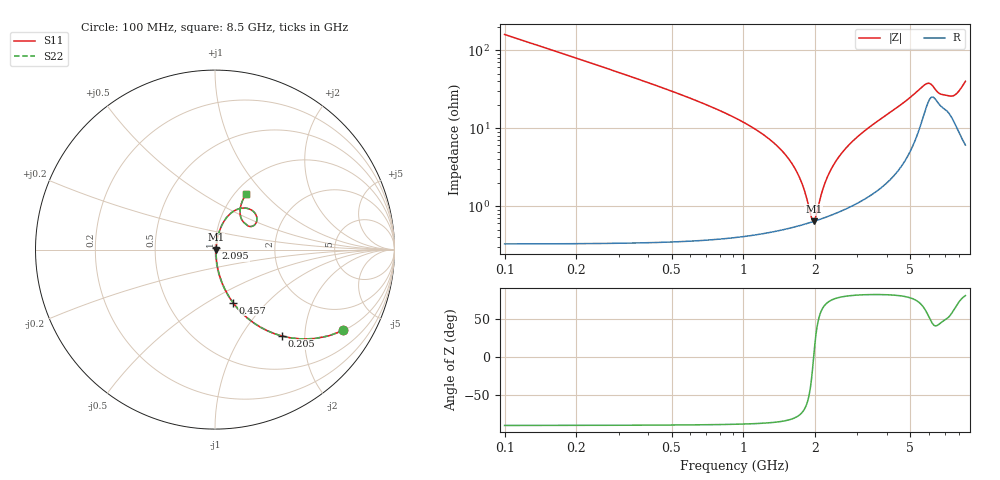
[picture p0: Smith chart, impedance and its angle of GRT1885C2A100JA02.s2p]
!Murata Part Number: GRT1885C2A100JA02
!These Parameters are Measured in Series Mode Connection
!Data Generated on Jun 19, 2026
!  o--ll--o
!Port1  Port2
!  o------o
!Operation Temp=25[degC], DC Bias Voltage=0[V]
!Freq. Start=100[MHz] Stop=9[GHz] 401[Steps]
# Hz S RI R 50
!Freq.(Hz) S11(Real) S11(Imag) S21(Real) S21(Imag) S12(Real) S12(Imag) S22(Real) S22(Imag)
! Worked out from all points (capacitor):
!   401 points, 100 MHz to 8.5 GHz, reference 50 ohm
!   read as one part in series: C = 10 pF near 142 MHz
!   lowest |Z| = 637 mohm at 1.969 GHz (marker M1)
!   series resonance near 1.968 GHz, so ESL is about 650 pH
!   S11 on the Smith chart (normalised r, x): 100 MHz: 1.01, -3.18; 205 MHz: 1.01, -1.54; 457 MHz: 1.01, -0.66; 2.095 GHz: 1.01, +0.02; 8.5 GHz: 1.12, +0.79
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1e8  0.7155 -0.4501  0.2845 0.4501  0.2845 0.4501  0.7155 -0.4501
2.05e8  0.3717 -0.4811  0.6283 0.4811  0.6283 0.4811  0.3717 -0.4811
3.1e8  0.2023 -0.3984  0.7977 0.3984  0.7977 0.3984  0.2023 -0.3984
4.57e8  0.1007 -0.2958  0.8993 0.2958  0.8993 0.2958  0.1007 -0.2958
8.56e8  0.0261 -0.1471  0.9739 0.1471  0.9739 0.1471  0.0261 -0.1471
1.507e9  0.007 -0.0439  0.993 0.0439  0.993 0.0439  0.007 -0.0439
1.717e9  0.0061 -0.0224  0.9939 0.0224  0.9939 0.0224  0.0061 -0.0224
1.927e9  0.00621 -0.00345  0.9938 0.00345  0.9938 0.00345  0.00621 -0.00345
1.969e9  0.00633 0.000106  0.9937 -0.000106  0.9937 -0.000106  0.00633 0.000106
2.011e9  0.00648 0.00359  0.9935 -0.00359  0.9935 -0.00359  0.00648 0.00359
2.095e9  0.00685 0.0104  0.9931 -0.0104  0.9931 -0.0104  0.00685 0.0104
2.221e9  0.0076 0.0202  0.9924 -0.0202  0.9924 -0.0202  0.0076 0.0202
2.389e9  0.0089 0.0327  0.9911 -0.0327  0.9911 -0.0327  0.0089 0.0327
2.914e9  0.0151 0.0688  0.9849 -0.0688  0.9849 -0.0688  0.0151 0.0688
3.481e9  0.0256 0.1058  0.9744 -0.1058  0.9744 -0.1058  0.0256 0.1058
4.3e9  0.0517 0.1604  0.9483 -0.1604  0.9483 -0.1604  0.0517 0.1604
5.707e9  0.1941 0.225  0.8059 -0.225  0.8059 -0.225  0.1941 0.225
6.001e9  0.2317 0.1847  0.7683 -0.1847  0.7683 -0.1847  0.2317 0.1847
6.358e9  0.213 0.1323  0.787 -0.1323  0.787 -0.1323  0.213 0.1323
7.114e9  0.1675 0.1455  0.8325 -0.1455  0.8325 -0.1455  0.1675 0.1455
7.702e9  0.1417 0.1878  0.8583 -0.1878  0.8583 -0.1878  0.1417 0.1878
8.5e9  0.1714 0.3076  0.8286 -0.3076  0.8286 -0.3076  0.1714 0.3076
